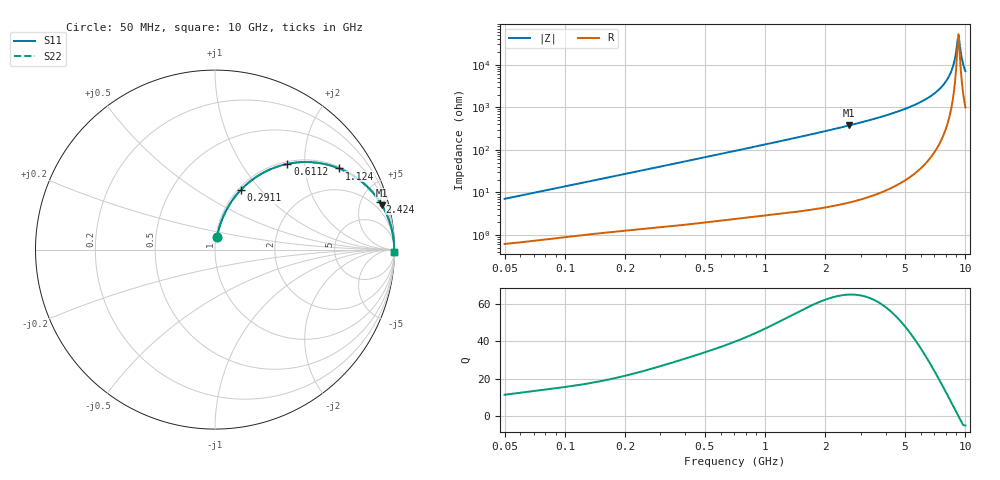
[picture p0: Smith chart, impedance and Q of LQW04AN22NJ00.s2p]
!Murata Part Number: LQW04AN22NJ00
!These Parameters are Measured in Series Mode Connection
!  o--[Z]--o
!Port1  Port2
!  o-------o
!Freq. Start=50[MHz] Stop=10[GHz], 401[Steps]
# Hz S RI R 50
!Freq.(Hz)	S 11(Real)	S 11(Imag)	S 21(Real)	S 21(Imag)	S 12(Real)	S 12(Imag)	S 22(Real)	S 22(Imag)
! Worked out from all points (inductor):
!   401 points, 50 MHz to 10 GHz, reference 50 ohm
!   read as one part in series: L = 22.3 nH near 51.34 MHz
!   highest Q = 65.1 at 2.624 GHz (marker M1), where L = 22.7 nH
!   self-resonance near 9.114 GHz
!   S11 on the Smith chart (normalised r, x): 50 MHz: 1.01, +0.14; 291.1 MHz: 1.03, +0.78; 611.2 MHz: 1.04, +1.64; 1.124 GHz: 1.06, +3.02; 2.424 GHz: 1.11, +6.84; 10 GHz: open
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5e7  0.0109 0.0691  0.9891 -0.0691  0.9891 -0.0691  0.0109 0.0691
1.214486e8  0.0361 0.1593  0.9639 -0.1593  0.9639 -0.1593  0.0361 0.1593
2.911136e8  0.1428 0.3314  0.8572 -0.3314  0.8572 -0.3314  0.1428 0.3314
2.949953e8  0.1458 0.3345  0.8542 -0.3345  0.8542 -0.3345  0.1458 0.3345
6.112328e8  0.4033 0.4774  0.5967 -0.4774  0.5967 -0.4774  0.4033 0.4774
7.071068e8  0.4728 0.4869  0.5272 -0.4869  0.5272 -0.4869  0.4728 0.4869
1.124152e9  0.6913 0.452  0.3087 -0.452  0.3087 -0.452  0.6913 0.452
1.717543e9  0.8418 0.3566  0.1582 -0.3566  0.1582 -0.3566  0.8418 0.3566
2.423676e9  0.9177 0.2671  0.0823 -0.2671  0.0823 -0.2671  0.9177 0.2671
2.624158e9  0.9302 0.2472  0.0698 -0.2472  0.0698 -0.2472  0.9302 0.2472
4.171863e9  0.9767 0.1423  0.0233 -0.1423  0.0233 -0.1423  0.9767 0.1423
5.965537e9  0.9923 0.0747  0.00769 -0.0747  0.00769 -0.0747  0.9923 0.0747
7.472112e9  0.9968 0.0359  0.00321 -0.0359  0.00321 -0.0359  0.9968 0.0359
7.983737e9  0.9975 0.0247  0.00252 -0.0247  0.00252 -0.0247  0.9975 0.0247
8.418147e9  0.9978 0.0157  0.00216 -0.0157  0.00216 -0.0157  0.9978 0.0157
8.759398e9  0.998 0.00895  0.00199 -0.00895  0.00199 -0.00895  0.998 0.00895
8.994549e9  0.9981 0.00443  0.00194 -0.00443  0.00194 -0.00443  0.9981 0.00443
9.114482e9  0.9981 0.00216  0.00193 -0.00216  0.00193 -0.00216  0.9981 0.00216
9.236013e9  0.9981 -0.000109  0.00193 0.000109  0.00193 0.000109  0.9981 -0.000109
9.359165e9  0.9981 -0.00239  0.00194 0.00239  0.00194 0.00239  0.9981 -0.00239
9.738562e9  0.998 -0.00928  0.00205 0.00928  0.00205 0.00928  0.998 -0.00928
1e10  0.9978 -0.0139  0.00218 0.0139  0.00218 0.0139  0.9978 -0.0139
